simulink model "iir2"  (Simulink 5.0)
settings: Solver=ode45  StartTime=0.0  StopTime=0.1  MaxStep=1e-5  RelTol=1e-3
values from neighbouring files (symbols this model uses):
  a1 = nenner(1,:,2)    [iir_2.m]
  a2 = nenner(2,:,2)    [iir_2.m]
  a3 = nenner(3,:,2)    [iir_2.m]
  a4 = nenner(5,:,2)    [iir_2.m]
  a5 = nenner(4,:,2)    [iir_2.m]
  b1 = (2*fr)*sin(2*pi*fr*k+eps)./(2*pi*fr*k+eps)    [fir_fenster1.m]    (also in iir_2.m = zaehler(1,:,2); TP_fdesign1.m = b1*prod(H1.ScaleValues); TP_fdesign2.m = H1.Numerator)
  b2 = b1.*w_fenster    [fir_fenster1.m]    (also in iir_2.m = zaehler(2,:,2); TP_fdesign1.m = H2.Numerator)
  b3 = zaehler(3,:,2)    [iir_2.m]
  b4 = zaehler(5,:,2)    [iir_2.m]
  b5 = zaehler(4,:,2)    [iir_2.m]
  f1 = 100    [ein_seiten_1.m]    (also in ein_seiten_2.m; iir_2.m = ',num2str(f2),'Hz; quadratur_mod_1.m; analog_bp1.m = ',num2str(f1),' Hz)
  f2 = 400    [ein_seiten_1.m]    (also in ein_seiten_2.m; iir_2.m = 300; quadratur_mod_1.m = ',num2str(f2),' Hz']); analog_bp1.m = ',num2str(f2),' Hz)']))
  f3 = ',         num2str(f3),'Hz    [iir_2.m]    (also in analog_tp2.m = 500)
  frausch = 100    [fir_vergleich1.m]    (also in iir_2.m = ',   num2str(frausch),'Hz; analog_bp3.m = 250; analog_tp2.m = 500; noise_alias_.m = ',num2str(frausch),' Hz)']))
  frechteck = 10    [iir_2.m]    (also in analog_tp2.m = 20)
  fs = 8000    [differenzier_1.m]    (also in ein_seiten_1.m = 1000; ein_seiten_2.m = 1000; firpm_ord1.m; fir_fenster1.m = 1000)
  k = -22:22    [fir_fenster1.m]
  k1 = 1    [iir_2.m]    (also in analog_bp3.m = 0; einh_puls1.m = 0)
  k2 = 1    [iir_2.m]    (also in analog_bp3.m; einh_puls1.m)
  k3 = 1    [iir_2.m]    (also in analog_bp3.m)
  k4 = 0    [iir_2.m]    (also in analog_bp3.m)
  k5 = 0    [iir_2.m]
  kr = 0    [iir_2.m]
libraries: dspsigops x1, dsparch4 x1

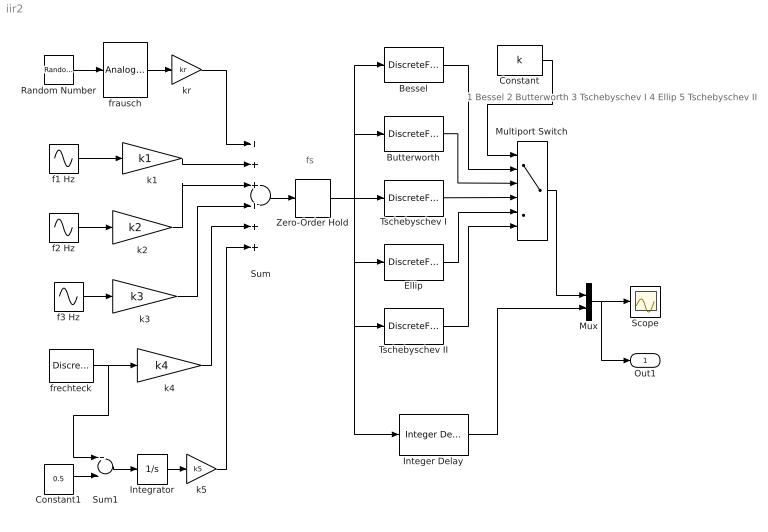
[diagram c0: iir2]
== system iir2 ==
  note: 1 Bessel 2 Butterworth 3 Tschebyschev I 4 Ellip 5 Tschebyschev II
  note: fs
  Bessel : DiscreteFilter  Numerator=[b1]  Denominator=[a1]  SampleTime=1/fs
  Butterworth : DiscreteFilter  Numerator=[b2]  Denominator=[a2]  SampleTime=1/fs
  Constant : Constant  Value=k
  Constant1 : Constant  Value=0.5
  Ellip : DiscreteFilter  Numerator=[b4]  Denominator=[a4]  SampleTime=1/fs
  Integer Delay : dspsigops/Integer Delay  delay=delay  ic=0  reset_popup=None
  Integrator : Integrator
  Multiport Switch : MultiPortSwitch  Inputs=5
  Mux : Mux  Inputs=2
  Random Number : RandomNumber  SampleTime=0
  Scope : Scope
  Sum : Sum  Inputs=++++++
  Sum1 : Sum  Inputs=+-
  Tschebyschev I : DiscreteFilter  Numerator=[b3]  Denominator=[a3]  SampleTime=1/fs
  Tschebyschev II : DiscreteFilter  Numerator=[b5]  Denominator=[a5]  SampleTime=1/fs
  Zero-Order Hold : ZeroOrderHold  SampleTime=1/fs
  f1 Hz : Sin  Frequency=2*pi*f1  SampleTime=0
  f2 Hz : Sin  Amplitude=1/3  Frequency=2*pi*f2  SampleTime=0
  f3 Hz : Sin  Amplitude=1/5  Frequency=2*pi*f3  SampleTime=0
  frausch : dsparch4/Analog Filter Design  method=Butterworth  filttype=Lowpass  N=8  Wlo=2*pi*frausch  Whi=80  Rp=2  Rs=40
  frechteck : DiscretePulseGenerator  PulseType=Time based  Period=1/frechteck  PulseWidth=50
  k1 : Gain  Gain=k1
  k2 : Gain  Gain=k2
  k3 : Gain  Gain=k3
  k4 : Gain  Gain=k4
  k5 : Gain  Gain=k5
  kr : Gain  Gain=kr
  Out1 : Outport
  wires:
  Random Number/1 -> frausch/1
  f1 Hz/1 -> k1/1
  f2 Hz/1 -> k2/1
  f3 Hz/1 -> k3/1
  kr/1 -> Sum/1
  k1/1 -> Sum/2
  k2/1 -> Sum/3
  k3/1 -> Sum/4
  Sum/1 -> Zero-Order Hold/1
  Bessel/1 -> Multiport Switch/2
  Butterworth/1 -> Multiport Switch/3
  Tschebyschev I/1 -> Multiport Switch/4
  Ellip/1 -> Multiport Switch/5
  Tschebyschev II/1 -> Multiport Switch/6
  Constant/1 -> Multiport Switch/1
  Mux/1 -> Scope/1, Out1/1
  Integer Delay/1 -> Mux/2
  frausch/1 -> kr/1
  frechteck/1 -> k4/1, Sum1/1
  Integrator/1 -> k5/1
  Sum1/1 -> Integrator/1
  Constant1/1 -> Sum1/2
  k4/1 -> Sum/5
  k5/1 -> Sum/6
  Zero-Order Hold/1 -> Bessel/1, Butterworth/1, Tschebyschev II/1, Integer Delay/1, Ellip/1, Tschebyschev I/1
  Multiport Switch/1 -> Mux/1
